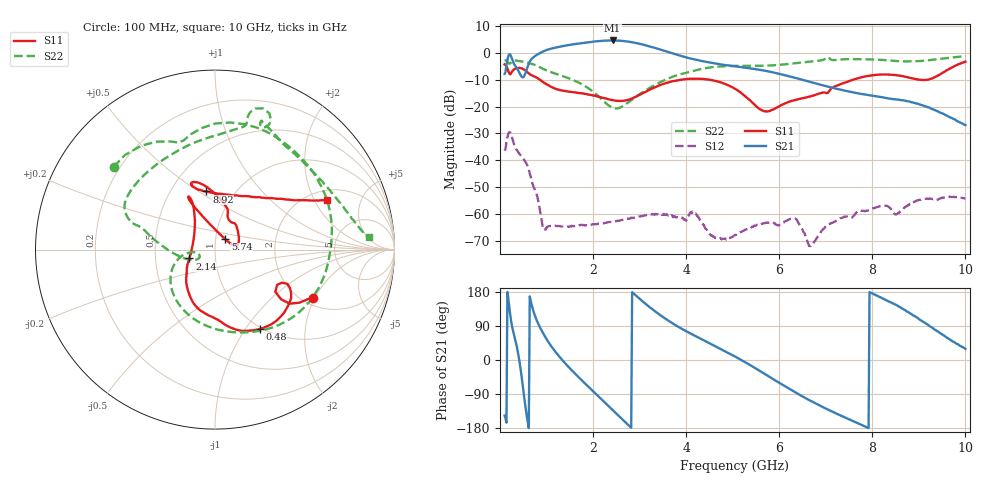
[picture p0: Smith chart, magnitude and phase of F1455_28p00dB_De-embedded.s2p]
! Integrated Device Technology
! Corporate Headquarters
! 6024 Silver Creek Valley Road
! San Jose, CA 95138  USA
! Phone:  1-408-284-8200
! Toll Free:  1-800-223-1366
! Webpage:  http://www.idt.com/
! Timing and RF Division
! 515 Groton Road, Suite 102
! Westford, MA 01886-6024
! Device:  F1455
! Description: 6-bit 0.5 dB Transmit Variable Gain Amplifier
! Frequency:  1400.0 -  2300.00 MHz
! Package:  6x6 mm Thin QFN Plastic Package: 28 pin
! State:  56
! Atten State:  28.0 dB
! Voltage:  +5.00 Volts
! Current:  217.626 mA
! Data:  The device was measured on a the F1455 evaluation board which has
!  individual transmission lines to the RF pins.  Data was collected
!  using a calibrated network analyzer.  The evaluation board was
!  de-embedded using a TRL calibration technique.
!  The reference plane is the edge of the package pin.
!  Pin  1 = CSb
!  Pin  2 = DATA
!  Pin  3 = CLK
!  Pin  4 = RSET
!  Pin  5 = GND
!  Pin  6 = RFIN  = Port 1
!  Pin  7 = GND
!  Pin  8 = NC
!  Pin  9 = NC
!  Pin 10 = NC
!  Pin 11 = NC
!  Pin 12 = NC
!  Pin 13 = NC
!  Pin 14 = /STBY
!  Pin 15 = GND
!  Pin 16 = RFOUT  = Port 2
!  Pin 17 = GND
!  Pin 18 = NC
!  Pin 19 = NC
!  Pin 20 = NC
!  Pin 21 = GND
!  Pin 22 = NC
!  Pin 23 = GND
!  Pin 24 = NC
!  Pin 25 = NC
!  Pin 26 = NC
!  Pin 27 = GND
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# GHz S dB R 50
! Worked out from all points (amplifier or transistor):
!   496 points, 100 MHz to 10 GHz, reference 50 ohm
!   highest |S21| = 4.6 dB at 2.42 GHz (marker M1)
!   |S21| within 3 dB of that: 1.113 GHz to 3.374 GHz (2.261 GHz wide, 101 % of centre)
!   unconditionally stable (mu >= 1): start of sweep to end of sweep
!   at 1.74 GHz: K = 472.53, MAG = 4.0 dB, |S12| = -64.0 dB
!   at 5.06 GHz: K = 1406.52, MAG = -3.1 dB, |S12| = -67.8 dB
!   at 10 GHz: K = 756.98, MAG = -18.2 dB, |S12| = -54.1 dB
!   S11 on the Smith chart (normalised r, x): 100 MHz: 2.27, -1.94; 480 MHz: 0.98, -1.17; 2.14 GHz: 0.75, -0.07; 5.74 GHz: 1.11, +0.13; 8.92 GHz: 0.74, +0.54; 10 GHz: 2.43, +2.56
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0.1  -4.29 -26.1  -7.87 -146.7  -36.39 47.7  -2.75 140.7
0.18  -6.71 -37.0  -1.25 161.4  -30.10 -6.3  -3.72 112.4
0.26  -6.99 -25.3  -2.25 88.9  -31.61 -77.3  -3.33 96.1
0.38  -5.65 -42.6  -6.17 24.4  -36.67 -118.9  -2.97 58.1
0.48  -5.87 -60.6  -9.12 -57.7  -38.93 -150.5  -3.23 31.4
0.66  -8.18 -88.0  -2.72 156.2  -46.20 140.3  -4.02 -11.0
0.78  -9.11 -103.1  -0.88 107.8  -52.28 116.3  -4.70 -37.8
0.94  -11.06 -121.8  0.60 67.8  -65.94 119.5  -6.09 -68.2
1.32  -13.98 -141.8  2.41 2.6  -64.61 119.7  -8.51 -119.1
1.76  -15.07 -151.2  3.63 -53.9  -64.03 88.6  -11.69 -155.9
2.14  -16.43 -161.0  4.40 -98.7  -63.59 74.4  -16.52 -173.1
2.42  -17.60 -176.9  4.60 -131.9  -62.88 66.9  -20.48 -164.9
2.82  -17.11 146.5  3.99 -178.7  -61.36 57.0  -17.66 -154.0
3.4  -12.28 118.6  1.46 122.3  -59.97 34.3  -11.33 178.8
4.08  -9.66 116.1  -2.05 71.0  -59.64 19.8  -7.11 162.9
5.06  -13.47 111.8  -5.03 8.6  -67.79 38.4  -4.85 147.9
5.74  -21.82 45.1  -6.82 -40.6  -63.15 31.5  -4.76 119.8
6.34  -17.55 14.0  -9.30 -84.9  -61.66 -13.6  -3.92 89.4
6.7  -16.08 34.4  -11.00 -109.5  -71.27 -168.1  -3.19 78.4
8.36  -8.08 109.5  -17.03 154.1  -57.44 66.0  -2.82 62.4
8.92  -9.70 98.3  -18.67 115.1  -55.34 79.5  -3.15 40.0
10  -3.29 24.0  -26.89 29.5  -54.08 12.9  -1.28 4.6
